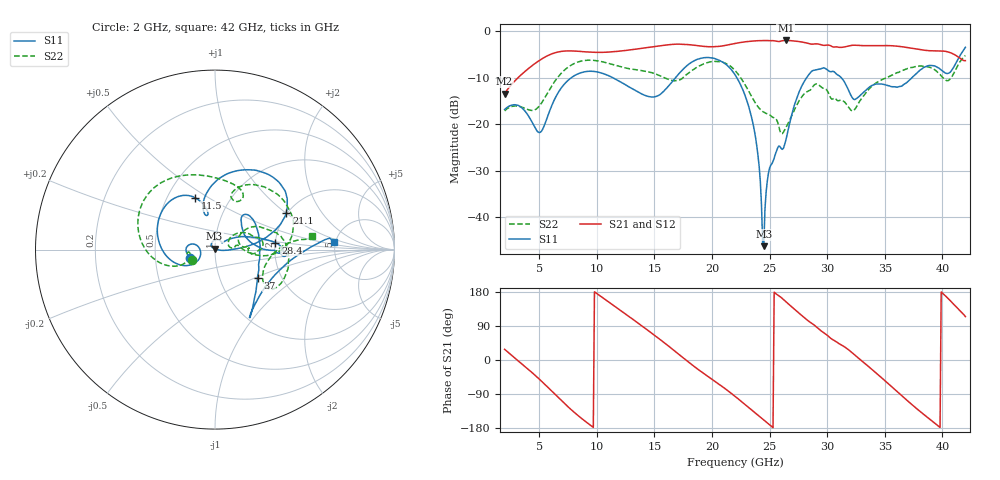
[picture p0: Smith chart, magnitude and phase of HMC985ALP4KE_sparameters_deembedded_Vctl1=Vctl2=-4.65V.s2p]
!s2p File: Measurements: S11, S21, S12, S22
# GHz S dB R 50.0
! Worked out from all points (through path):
!   401 points, 2 GHz to 42 GHz, reference 50 ohm
!   highest |S21| = -2.06 dB at 26.4 GHz (marker M1); lowest = -13.4 dB at 2 GHz (marker M2)
!   lowest |S11| = -46.1 dB at 24.5 GHz (marker M3), VSWR 1.01, Z = 49.8 + j0.447 ohm
!   |S11| at or under -10 dB: start of sweep to 7.817 GHz; 22.15 GHz to 28.23 GHz (6.082 GHz wide, 24.1 % of centre); 31.21 GHz to 37.38 GHz (6.169 GHz wide, 18 % of centre)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
!   |S22| runs from -22.0 to -5.3 dB; largest |S21 - S12| = 0.00069
!   S11 on the Smith chart (normalised r, x): 2 GHz: 0.76, -0.07; 11.5 GHz: 0.69, +0.44; 21.1 GHz: 1.97, +1.02; 28.4 GHz: 2.00, +0.18; 37 GHz: 1.51, -0.53; 42 GHz: 4.87, +0.75
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2  -16.85 -161.8  -13.43 28.2  -13.44 28.2  -17.15 -155.6
5  -21.80 -172.9  -6.38 -50.2  -6.38 -50.2  -16.15 -160.0
6.3  -14.86 -150.5  -4.76 -88.4  -4.76 -88.4  -11.02 -161.8
8.7  -8.92 150.3  -4.44 -154.6  -4.44 -154.6  -6.46 151.2
11.5  -10.18 111.0  -4.47 143.0  -4.47 143.0  -7.31 104.9
13.6  -13.14 101.3  -3.85 97.0  -3.85 97.0  -8.41 75.5
15.4  -13.80 106.1  -3.25 56.3  -3.25 56.3  -9.53 62.0
17.9  -7.31 80.1  -2.94 -3.8  -2.94 -3.8  -9.18 72.0
21.1  -6.98 27.4  -3.15 -74.6  -3.15 -74.6  -6.88 15.8
22  -9.39 16.9  -2.71 -95.8  -2.71 -95.8  -8.48 0.4
23.6  -20.34 0.3  -2.18 -135.6  -2.18 -135.5  -14.78 -4.3
24.5  -46.14 114.4  -2.08 -158.2  -2.08 -158.2  -17.42 8.4
25  -29.40 131.0  -2.11 -171.0  -2.10 -171.0  -17.99 11.2
26.4  -23.56 41.6  -2.06 154.3  -2.06 154.3  -20.85 33.0
28.4  -9.41 6.6  -2.72 102.3  -2.72 102.3  -12.86 18.1
28.7  -8.59 1.7  -2.86 96.1  -2.86 96.1  -12.18 16.2
30.7  -8.98 -3.3  -3.45 50.3  -3.45 50.3  -14.45 2.0
32.5  -14.59 32.3  -3.10 10.4  -3.10 10.4  -16.46 27.9
35.4  -11.80 18.9  -3.17 -65.1  -3.17 -65.1  -9.78 19.2
37  -10.88 -34.0  -3.59 -108.2  -3.59 -108.2  -8.06 4.7
39.8  -8.17 -57.2  -4.30 -177.9  -4.29 -177.9  -9.36 -35.7
42  -3.53 3.7  -6.39 114.4  -6.40 114.4  -5.28 8.2
